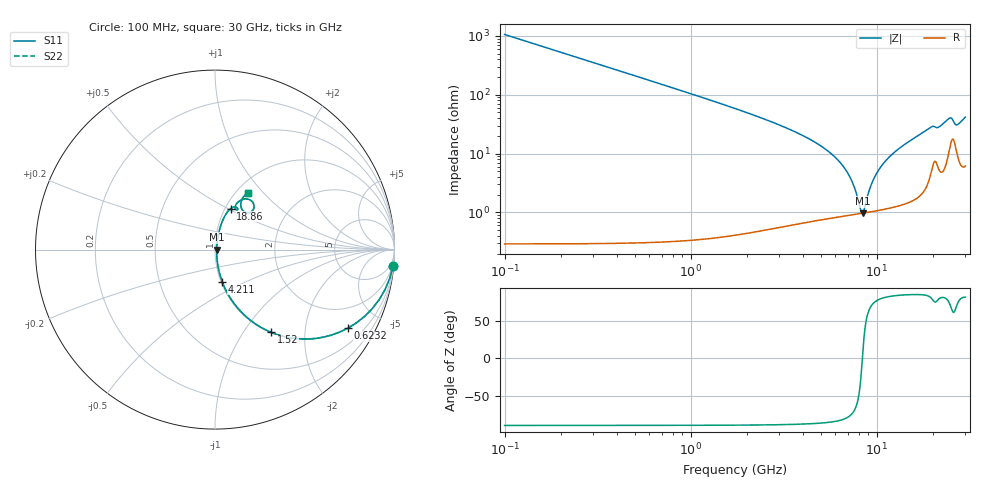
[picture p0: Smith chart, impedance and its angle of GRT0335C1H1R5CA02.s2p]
!Murata Part Number: GRT0335C1H1R5CA02
!These Parameters are Measured in Series Mode Connection
!Data Generated on Jun 19, 2026
!  o--ll--o
!Port1  Port2
!  o------o
!Operation Temp=25[degC], DC Bias Voltage=0[V]
!Freq. Start=100[MHz] Stop=30[GHz] 401[Steps]
# Hz S RI R 50
!Freq.(Hz) S11(Real) S11(Imag) S21(Real) S21(Imag) S12(Real) S12(Imag) S22(Real) S22(Imag)
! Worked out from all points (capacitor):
!   401 points, 100 MHz to 30 GHz, reference 50 ohm
!   read as one part in series: C = 1.5 pF near 249.5 MHz
!   lowest |Z| = 969 mohm at 8.397 GHz (marker M1)
!   series resonance near 8.381 GHz, so ESL is about 240 pH
!   S11 on the Smith chart (normalised r, x): 100 MHz: 1, -21; 623.2 MHz: 1.01, -3.38; 1.52 GHz: 1.01, -1.35; 4.211 GHz: 1.01, -0.37; 18.86 GHz: 1.06, +0.52; 30 GHz: 1.12, +0.83
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1e8  0.9912 -0.0934  0.00883 0.0934  0.00883 0.0934  0.9912 -0.0934
3.99e8  0.8753 -0.3298  0.1247 0.3298  0.1247 0.3298  0.8753 -0.3298
6.2325e8  0.7408 -0.4373  0.2592 0.4373  0.2592 0.4373  0.7408 -0.4373
9.97e8  0.5234 -0.4979  0.4766 0.4979  0.4766 0.4979  0.5234 -0.4979
1.52025e9  0.313 -0.4609  0.687 0.4609  0.687 0.4609  0.313 -0.4609
2.56675e9  0.1254 -0.3244  0.8746 0.3244  0.8746 0.3244  0.1254 -0.3244
4.21125e9  0.0398 -0.1783  0.9602 0.1783  0.9602 0.1783  0.0398 -0.1783
5.10825e9  0.0236 -0.1255  0.9764 0.1255  0.9764 0.1255  0.0236 -0.1255
6.977e9  0.0108 -0.0455  0.9892 0.0455  0.9892 0.0455  0.0108 -0.0455
7.575e9  0.00973 -0.025  0.9903 0.025  0.9903 0.025  0.00973 -0.025
8.24775e9  0.00951 -0.00397  0.9905 0.00397  0.9905 0.00397  0.00951 -0.00397
8.39725e9  0.00959 0.000475  0.9904 -0.000475  0.9904 -0.000475  0.00959 0.000475
9.29425e9  0.0108 0.0257  0.9892 -0.0257  0.9892 -0.0257  0.0108 0.0257
1.01165e10  0.0128 0.0469  0.9872 -0.0469  0.9872 -0.0469  0.0128 0.0469
1.206e10  0.0206 0.0922  0.9794 -0.0922  0.9794 -0.0922  0.0206 0.0922
1.505e10  0.0394 0.1542  0.9606 -0.1542  0.9606 -0.1542  0.0394 0.1542
1.886225e10  0.0873 0.2284  0.9127 -0.2284  0.9127 -0.2284  0.0873 0.2284
2.005825e10  0.1214 0.2347  0.8786 -0.2347  0.8786 -0.2347  0.1214 0.2347
2.245025e10  0.1215 0.2572  0.8785 -0.2572  0.8785 -0.2572  0.1215 0.2572
2.50665e10  0.2144 0.2567  0.7856 -0.2567  0.7856 -0.2567  0.2144 0.2567
2.678575e10  0.1573 0.2158  0.8427 -0.2158  0.8427 -0.2158  0.1573 0.2158
3e10  0.1819 0.3181  0.8181 -0.3181  0.8181 -0.3181  0.1819 0.3181
